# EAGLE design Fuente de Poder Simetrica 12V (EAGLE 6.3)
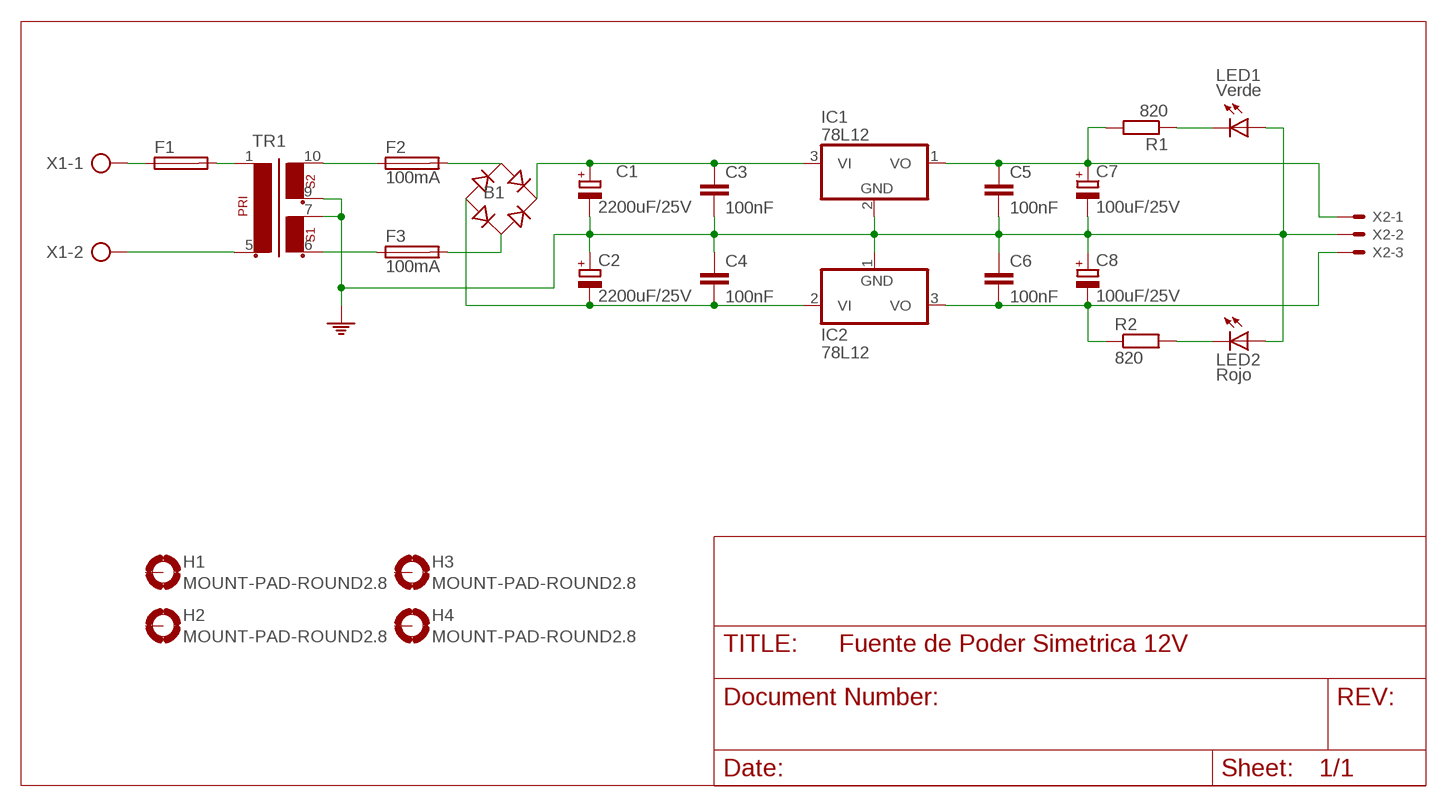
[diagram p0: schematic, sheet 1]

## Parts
B1  RB1A  [RB1A]
C1  2200uF/25V  CPOL-EUE2-5  [E2-5]
C2  2200uF/25V  CPOL-EUE2-5  [E2-5]
C3  100nF  C-EU050-025X075  [C050-025X075]
C4  100nF  C-EU050-025X075  [C050-025X075]
C5  100nF  C-EU050-025X075  [C050-025X075]
C6  100nF  C-EU050-025X075  [C050-025X075]
C7  100uF/25V  CPOL-EUE5-13  [E5-13]
C8  100uF/25V  CPOL-EUE5-13  [E5-13]
F1  19560  [19560]
F2  100mA  19560  [19560]
F3  100mA  19560  [19560]
H1  MOUNT-PAD-ROUND2.8  [2,8-PAD]
H2  MOUNT-PAD-ROUND2.8  [2,8-PAD]
H3  MOUNT-PAD-ROUND2.8  [2,8-PAD]
H4  MOUNT-PAD-ROUND2.8  [2,8-PAD]
IC1  78L12  78L12Z  [TO92]
IC2  78L12  79L12Z  [TO92]
LED1  Verde  TLLG4400  [LED3MM]
LED2  Rojo  TLLG4400  [LED3MM]
R1  820  R-EU_0204/7  [0204/7]
R2  820  R-EU_0204/7  [0204/7]
TR1  EI30-2  [EI30-2]
X1  AK300/2  [AK300/2]
X2  KK-156-3  [KK-156-3]

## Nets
GND: C1.- C2.+ C3.2 C4.1 C5.2 C6.1 C7.- C8.+ IC1.2(GND) IC2.1(GND) LED1.A LED2.A TR1.7 TR1.9 X2.2
N$1: F1.1 X1.1
N$2: F1.2 TR1.1
N$3: TR1.5 X1.2
N$4: F2.1 TR1.10
N$5: B1.AC1 F2.2
N$6: B1.AC2 F3.2
N$7: F3.1 TR1.6
N$8: B1.+ C1.+ C3.1 IC1.3(VI)
N$9: C5.1 C7.+ IC1.1(VO) R1.2 X2.1
N$10: LED1.K(C) R1.1
N$11: B1.- C2.- C4.2 IC2.2(VI)
N$12: C6.2 C8.- IC2.3(VO) R2.1 X2.3
N$13: LED2.K(C) R2.2
Unconnected: H1.B2,8(MOUNT) H2.B2,8(MOUNT) H3.B2,8(MOUNT) H4.B2,8(MOUNT)

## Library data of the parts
B1 = rectifier:RB1A: RECTIFIER 1 A
C1 C2 C7 C8 = rcl:CPOL-EU: POLARIZED CAPACITOR, European symbol
C3-C6 = rcl:C-EU: CAPACITOR, European symbol
F1-F3 = fuse:19560: FUSE HOLDER; MPN: 56000001009; OC_FARNELL: 1185363; OC_NEWARK: 15P8392
H1-H4 = holes:MOUNT-PAD-ROUND: MOUNTING PAD, round
IC1 = linear:78*: Positive VOLTAGE REGULATOR Source: http://cache.national.com/ds/LM/LM78L05.pdf http://www.fairchildsemi.com/ds/LM/LM7805.pdf
IC2 = linear:79*: Negative VOLTAGE REGULATOR
LED1 LED2 = led:TLLG4400: Low Current (2mA) LED 3 mm Tinted Diffused Package color GREEN; MF: VISHAY SEMICONDUCTOR; OC_FARNELL: 1612435
R1 R2 = rcl:R-EU_: RESISTOR, European symbol
TR1 = trafo:EI30-2: TRANSFORMER 1 primary winding, 2 secondary windings ERA
X1 = con-ptr500:AK300/2: CONNECTOR; OC_FARNELL: unknown; OC_NEWARK: unknown
X2 = con-molex:KK-156-3: KK 156 HEADER Source: http://www.molex.com/pdm_docs/sd/026604100_sd.pdf; OC_FARNELL: unknown; OC_NEWARK: unknown

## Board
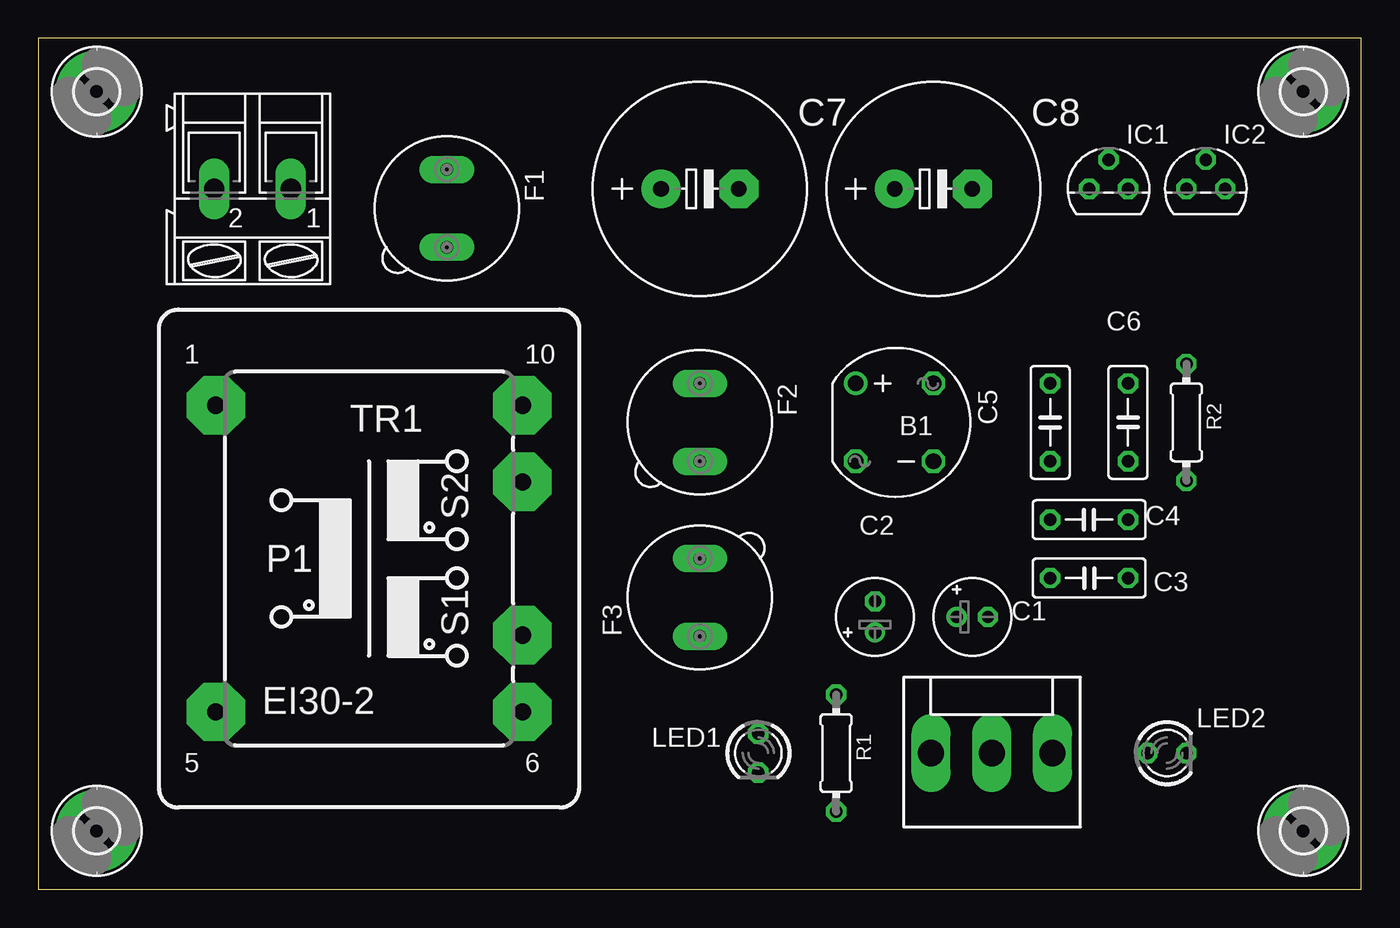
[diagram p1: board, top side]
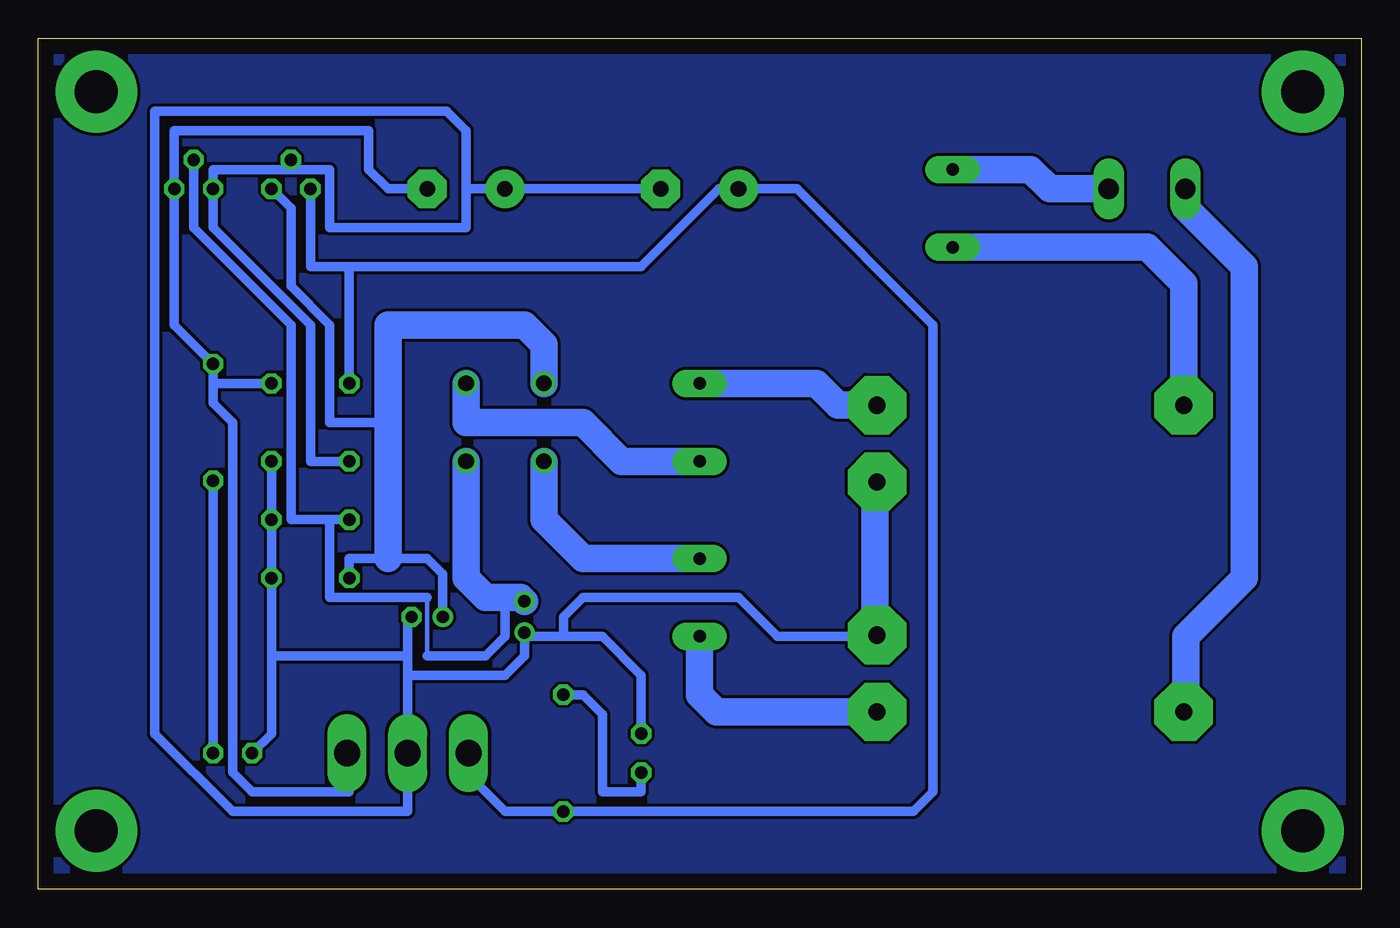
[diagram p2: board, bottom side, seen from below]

Size 86.34 x 55.55 mm. Coordinates in mm from the lower left corner, seen from the top.
Outline: 0,0 86.34,0 86.34,55.55 0,55.55 0,0
Copper layers (1*16): Top 0.035mm / dielectric 1.5mm / Bottom 0.035mm
Design rules "default": minimum track width 10mil, minimum drill 24mil, track to track 8mil, track to pad 8mil, pad to pad 8mil, via to via 8mil, smd to smd 8mil, copper to edge 40mil, drill to drill 8mil, minimum pad ring 10mil, minimum via ring 8mil, stop-mask expansion 4mil, vias tented up to drill 0mil, thermal gap 10mil

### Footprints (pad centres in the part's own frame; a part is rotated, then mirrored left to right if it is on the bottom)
RB1A = drill 1.016: + -2.54,2.54 | drill 1.016 octagon: - 2.54,-2.54; AC1 2.54,2.54; AC2 -2.54,-2.54
E2-5 = drill 0.813 pad 1.27: + -1.016,0 | drill 0.813 pad 1.27 octagon: - 1.016,0
C050-025X075 = drill 0.813 octagon: 1 -2.54,0; 2 2.54,0
E5-13 = drill 1.016 pad 2.54: + -2.54,0 | drill 1.016 pad 2.54 octagon: - 2.54,0
19560 = drill 0.813 pad 1.778 long: 1 -2.54,0; 2 2.54,0
2,8-PAD = drill 2.8 pad 5.334: B2,8 0,0
TO92 = drill 0.813 octagon: 1 -1.27,0; 2 0,1.905; 3 1.27,0
LED3MM = drill 0.813 octagon: A -1.27,0; K 1.27,0
0204/7 = drill 0.813 octagon: 1 -3.81,0; 2 3.81,0
EI30-2 = drill 1.118 pad 3.81 octagon: 1 -10.008,10.008; 5 -10.008,-10.008; 6 10.008,-10.008; 7 10.008,-5.004; 9 10.008,5.004; 10 10.008,10.008
AK300/2 = drill 1.321 long: 1 -2.515,0; 2 2.489,0
KK-156-3 = drill 1.7 pad 2.184 long: 1 -3.96,0; 2 0,0; 3 3.96,0

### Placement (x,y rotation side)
B1  55.88,30.48 0 top
C1  60.96,17.78 0 top
C2  54.61,17.78 90 top
C3  68.58,20.32 0 top
C4  68.58,24.13 180 top
C5  66.04,30.48 270 top
C6  71.12,30.48 90 top
C7  43.18,45.72 0 top
C8  58.42,45.72 0 top
F1  26.67,44.45 270 top
F2  43.18,30.48 270 top
F3  43.18,19.05 90 top
H1  MOUNT-HOLE2.8  [2,8-PAD]  3.81,3.81 0 top
H2  MOUNT-HOLE2.8  [2,8-PAD]  3.81,52.07 0 top
H3  MOUNT-HOLE2.8  [2,8-PAD]  82.55,3.81 0 top
H4  MOUNT-HOLE2.8  [2,8-PAD]  82.55,52.07 0 top
IC1  69.85,45.72 0 top
IC2  76.2,45.72 0 top
LED1  46.99,8.89 270 top
LED2  73.66,8.89 0 top
R1  52.07,8.89 270 top
R2  74.93,30.48 270 top
TR1  21.59,21.59 0 top
X1  120 VCA  [AK300/2]  13.97,45.72 180 top
X2  + - 12 VCD  [KK-156-3]  62.23,8.89 0 top

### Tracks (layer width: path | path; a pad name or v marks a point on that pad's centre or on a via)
GND
  Bottom 0.61: C7.- C8.+ 58.42,45.72 | C5.2 68.58,27.94 68.58,36.83 74.93,43.18 IC2.1 74.93,46.99 69.85,46.99 | 69.85,46.99 67.31,46.99 67.31,43.18 58.42,43.18 58.42,45.72 | 69.85,46.99 IC1.2 | LED2.A 71.12,10.16 71.12,15.24 | 71.12,15.24 C3.2 C4.1 C6.1 | 62.23,13.97 X2.2 62.23,5.08 73.66,5.08 78.74,10.16 78.74,50.8 59.69,50.8 58.42,49.53 58.42,45.72 | 62.23,13.97 62.23,15.24 | LED1.A 46.99,13.97 49.53,16.51 52.07,16.51 | 52.07,16.51 54.36,16.51 C2.+ 54.61,15.24 55.88,13.97 62.23,13.97 | 31.75,16.51 38.1,16.51 40.64,19.05 50.8,19.05 52.07,17.78 52.07,16.51 | 62.23,15.24 71.12,15.24 | 62.23,15.24 62.23,17.78 C1.-
  Bottom 1.778: TR1.9 31.75,26.44 31.75,16.51 31.67,16.51 TR1.7
N$1
  Bottom 1.778: F1.1 21.59,46.99 20.32,45.72 X1.1
N$2
  Bottom 1.778: TR1.1 11.58,39.52 13.97,41.91 F1.2
N$3
  Bottom 1.778: X1.2 11.48,44.5 7.62,40.64 7.62,20.32 11.43,16.51 11.43,11.73 TR1.5
N$4
  Bottom 1.778: TR1.10 34.14,31.6 35.56,33.02 F2.1
N$5
  Bottom 1.778: F2.2 48.26,27.94 50.8,30.48 58.42,30.48 B1.AC1
N$6
  Bottom 1.778: F3.2 50.8,21.59 53.34,24.13 B1.AC2
N$7
  Bottom 1.778: TR1.6 42.06,11.58 43.18,12.7 F3.1
N$8
  Bottom 0.61: IC1.3 69.85,44.45 69.85,39.37 67.31,36.83 67.31,30.48 63.5,30.48 | C1.+ 59.94,20.57 60.96,21.59 63.5,21.59 66.04,21.59 C3.1
  Bottom 1.778: B1.+ 53.34,35.56 54.61,36.83 63.5,36.83 63.5,30.48 63.5,21.59
N$9
  Bottom 0.61: X2.1 58.42,8.74 58.42,7.62 55.88,5.08 R1.2 29.21,5.08 27.94,6.35 27.94,36.83 36.83,45.72 C7.+ 41.91,45.72 46.99,40.64 66.04,40.64 | IC1.1 68.58,40.64 66.04,40.64 | 66.04,40.64 C5.1
N$10
  Bottom 0.61: LED1.K 46.99,6.35 49.53,6.35 49.53,11.43 50.8,12.7 R1.1
N$11
  Bottom 0.305: 60.96,19.05 60.96,15.24
  Bottom 0.61: 67.31,24.13 69.85,24.13 69.85,36.83 76.2,43.18 IC2.2 | 67.31,24.13 C4.2 | 60.96,19.05 67.31,19.05 67.31,24.13 | 60.96,15.24 57.15,15.24 55.88,16.51 55.88,19.05
  Bottom 1.778: B1.- 58.42,20.32 57.15,19.05 55.88,19.05 54.86,19.05 C2.-
N$12
  Bottom 0.61: 74.93,33.02 C6.2 | 74.93,33.02 R2.1 77.47,36.83 IC2.3 77.47,49.53 64.77,49.53 64.77,46.99 63.5,45.72 C8.- | 74.93,33.02 74.93,31.75 73.66,30.48 73.66,7.62 72.39,6.35 66.04,6.35 66.04,8.74 X2.3
N$13
  Bottom 0.61: R2.2 LED2.K
N$14
  pour Bottom: 60.96,55.88 86.36,55.88 86.36,0 0,0 0,55.88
